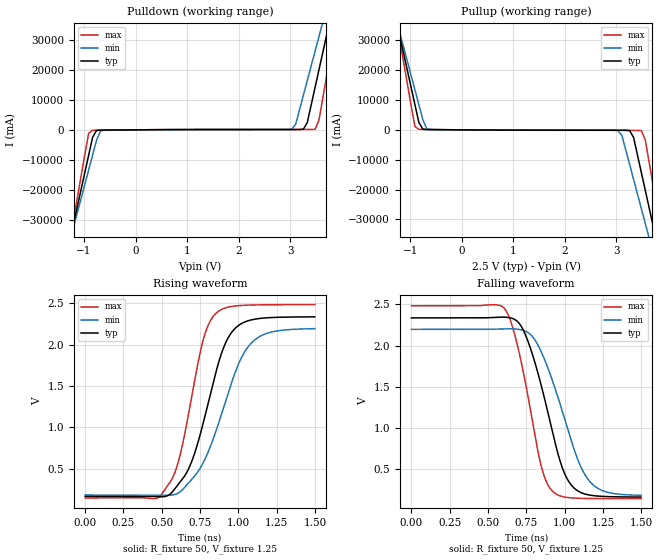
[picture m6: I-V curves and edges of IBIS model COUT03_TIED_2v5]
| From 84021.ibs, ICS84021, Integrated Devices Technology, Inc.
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[Model] COUT03_TIED_2v5
Model_type  Output
Polarity   Non-Inverting
Vmeas = 1.25
Rref = 50
Cref = 0
Vref = 1.25
|Variable  typ   min   max
C_comp   2p   1.5p   2.5p
[Voltage Range]   2.5   2.375   2.625
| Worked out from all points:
|   slope of the pulldown table from 0 to 0.375 V, typ, clamps not added: 8.25 ohm
|   slope of the pullup table from 0 to 0.375 V, typ, clamps not added: 8.09 ohm
|   rising waveform, R_fixture 50, V_fixture 1.25: 20-80 % time 193ps typ, 233ps min, 152ps max; typ from 0.163 V to 2.34 V
|   falling waveform, R_fixture 50, V_fixture 1.25: 20-80 % time 182ps typ, 215ps min, 147ps max; typ from 2.34 V to 0.164 V
| Open source, no load
|  Voltage   I(typ)   I(min)   I(max)
[Pullup]
-2.5V     132.6A     116.7A     159.5A
-1.288V   37.98A     37.97A     38.54A
-1.212V   32.07A     33.05A     30.99A
-909.1mV  8.434A     13.37A     1.158A
-833.3mV  2.525A     8.451A     173.9mA
-606.1mV  90.63mA    109.2mA    109.4mA
3.03V     -134.4mA   -266.8mA   -166.9mA
3.333V    -2.551A    -16.58A    -175.2mA
3.485V    -14.36A    -26.42A    -275mA
3.712V    -32.08A    -41.17A    -18.54A
3.864V    -43.9A     -51.01A    -33.65A
5V        -132.5A    -124.8A    -146.9A
[Pulldown]
-2.5V     -132.5A    -116.7A    -159.4A
-1.288V   -37.96A    -37.96A    -38.51A
-1.212V   -32.05A    -33.04A    -30.96A
-909.1mV  -8.418A    -13.36A    -1.131A
-833.3mV  -2.509A    -8.439A    -148.2mA
-606.1mV  -78.65mA   -99.19mA   -90.66mA
3.03V     104.5mA    238.1mA    123.5mA
3.333V    2.506A     16.54A     124.3mA
3.485V    14.31A     26.37A     211mA
3.712V    32.01A     41.11A     18.46A
3.864V    43.82A     50.94A     33.55A
5V        132.4A     124.7A     146.8A
[Ramp]
|   typ   min   max
dV/dt_r   1.742/0.307n   1.614/0.37n   1.879/0.24n
dV/dt_f   1.746/0.272n   1.616/0.322n   1.882/0.22n
R_load =   50.0000
[Rising Waveform]
R_fixture = 50
V_fixture = 1.25   | VCC_typ
V_fixture_max = 1.3125   | VCC_max
V_fixture_min = 1.1875   | VCC_min
C_fixture = 0.0p
| Time   typ   min   max
0s        162.8mV    179.2mV    144.2mV
459.5ps   160.6mV    180.1mV    137.1mV
546.5ps   180.2mV    176.8mV    312.4mV
614.1ps   322.8mV    210.7mV    623.9mV
696.7ps   592.1mV    370.8mV    1.384V
777.8ps   1.105V     597mV      2.106V
860.4ps   1.714V     990.7mV    2.39V
952ps     2.139V     1.519V     2.462V
1.087ns   2.301V     2.025V     2.48V
1.498ns   2.337V     2.194V     2.484V
[Falling Waveform]
R_fixture = 50
V_fixture = 1.25   | VCC_typ
V_fixture_max = 1.3125   | VCC_max
V_fixture_min = 1.1875   | VCC_min
C_fixture = 0.0p
| Time   typ   min   max
0s        2.337V     2.198V     2.484V
597.6ps   2.347V     2.205V     2.469V
671.2ps   2.321V     2.204V     2.155V
764.3ps   2.037V     2.154V     1.353V
833.3ps   1.616V     1.981V     651.8mV
878.4ps   1.287V     1.789V     360.6mV
968.5ps   612.6mV    1.304V     179.4mV
1.036ns   327.6mV    893.1mV    155.3mV
1.192ns   180.2mV    301.7mV    145.9mV
1.498ns   163.9mV    185mV      144.3mV
